| IBIS file usssdx1xxax.ibs created by s2ibis3 verion 1.1
| North Carolina State University, ERL, 2006
| This Model is valid for High-Rel grade Temperature Range -55C<=Tc<=125C
| Valid for DDR-333/400 operation
| Part Number   VDD/VDDQ   Package   Architecture
| SCB25D1G800AF   2.5 +0.2/-0.2  60-Ball FBGA   128Meg x 8
| SCB25D512800AF   2.5 +0.2/-0.2  60-Ball FBGA   64Meg x 8
| SCB25D1G160AF   2.5 +0.2/-0.2  60-Ball FBGA   64Meg x 16
| SCB25D1G160AE   2.5 +0.2/-0.2  66-Pin  Tsop   64Meg x 16
| SCB25D1G800AE   2.5 +0.2/-0.2  66-Pin  Tsop   128Meg x 8
| SCB25D512800AE   2.5 +0.2/-0.2  66-Pin  Tsop   64Meg x 8
| SCB25D512160AF   2.5 +0.2/-0.2  60-Ball FBGA   32Meg x 16
| SCB25D512160AE   2.5 +0.2/-0.2  66-Pin  Tsop   32Meg x 16
[IBIS Ver]   3.2
[File name]  usssdx1xxax.ibs
[File Rev]   1.2
[Date]   2016-10-27
[Source]   Simulation of a silicon level SPICE model
[Notes]   IBIS Characteristics for I/O Buffer
   IBIS Model Revision History:
Rev 1.1: 2015-10-27
   - IBIS model file initial creation
Rev 1.2: 2016-10-27
   - Updata company and other informations
   - Put components with different package into one IBIS model
[disclaimer] The IBIS models are for modeling purpose only and are
   subject to change without any notice. UniIC is not
   responsible for any problems the models may cause.
[Copyright]  Copyright 2009 UniIC Semiconductors Corp. All rights reserved
|   Component SCB25D1G800AF
[Component]   SCB25D1G800AF
[Manufacturer]  UniIC Semiconductors Corp.
| All balls excluding NC, POWER and GND (R[Ohm], L[H], C[F])
[Package]   |60-Ball FBGA
|Variable   typ   min   max
R_pkg   347m   219m   797m
L_pkg   1.51n   0.84n   3.21n
C_pkg   1.16p   0.74p   1.68p
[Pin]   signal_name model_name   R_pin   L_pin   C_pin
A1   VSSQ   GND
A2   DQ7   DQ   678m   2.88n   1.52p
A3   VSS   GND
A7   VDD   POWER
A8   DQ0   DQ   439m   1.68n   1.31p
A9   VDDQ   POWER
B2   VDDQ   POWER
B3   DQ6   DQ   797m   3.21n   1.68p
B7   DQ1   DQ   325m   1.24n   1.16p
B8   VSSQ   GND
C2   VSSQ   GND
C3   DQ5   DQ   476m   2.21n   1.25p
C7   DQ2   DQ   271m   0.99n   1.08p
C8   VDDQ   POWER
D2   VDDQ   POWER
D3   DQ4   DQ   395m   1.80n   1.16p
D7   DQ3   DQ   234m   0.84n   1.04p
D8   VSSQ   GND
E2   VSSQ   GND
E3   DQS   DQ   350m   1.48n   1.11p
E8   VDDQ   POWER
F1   VREF   POWER
F2   VSS   GND
F3   DM   DATA_RCV   299m   1.32n   1.04p
F8   VDD   POWER
F9   A5   CLKCA_RCV   314m   1.43n   1.13p
G2   CK   CLKCA_RCV   248m   1.16n   1.19p
G3   CK#   CLKCA_RCV   341m   1.59n   1.06p
G7   WE#   CLKCA_RCV   232m   1.10n   1.00p
G8   CAS#   CLKCA_RCV   340m   1.50n   1.18p
H2   A4   CLKCA_RCV   463m   1.90n   1.31p
H3   CKE   CLKCA_RCV   221m   1.03n   1.02p
H7   RAS#   CLKCA_RCV   219m   1.03n   1.01p
H8   CS#   CLKCA_RCV   318m   1.45n   1.14p
J2   A3   CLKCA_RCV   396m   1.83n   1.22p
J3   A13   CLKCA_RCV   438m   1.98n   1.29p
J7   BA1   CLKCA_RCV   242m   1.05n   1.06p
J8   BA0   CLKCA_RCV   357m   1.54n   1.21p
K2   A12   CLKCA_RCV   326m   1.52n   1.16p
K3   A11   CLKCA_RCV   340m   1.43n   1.18p
K7   A0   CLKCA_RCV   228m   1.03n   1.00p
K8   A2   CLKCA_RCV   264m   1.22n   1.08p
L2   A10   CLKCA_RCV   316m   1.49n   1.13p
L3   A9   CLKCA_RCV   236m   1.06n   1.02p
L7   A6   CLKCA_RCV   394m   1.66n   1.24p
L8   A1   CLKCA_RCV   344m   1.44n   1.19p
M2   A8   CLKCA_RCV   360m   1.57n   1.18p
M3   VSS   GND
M7   VDD   POWER
M8   A7   CLKCA_RCV   251m   1.04n   1.07p
|*****************************  Diff Pin  *************************************
[Diff Pin]  inv_pin  vdiff   tdelay_typ  tdelay_min  tdelay_max
G2   G3   0.62V   NA   NA   NA
|   Component SCB25D512800AF
[Component]   SCB25D512800AF
[Manufacturer]  UniIC Semiconductors Corp.
| All balls excluding NC, POWER and GND (R[Ohm], L[H], C[F])
[Package]   |60-Ball FBGA
|Variable   typ   min   max
R_pkg   347m   219m   797m
L_pkg   1.51n   0.84n   3.21n
C_pkg   1.16p   0.74p   1.68p
[Pin]   signal_name model_name   R_pin   L_pin   C_pin
A1   VSSQ   GND
A2   DQ7   DQ   678m   2.88n   1.52p
A3   VSS   GND
A7   VDD   POWER
A8   DQ0   DQ   439m   1.68n   1.31p
A9   VDDQ   POWER
B2   VDDQ   POWER
B3   DQ6   DQ   797m   3.21n   1.68p
B7   DQ1   DQ   325m   1.24n   1.16p
B8   VSSQ   GND
C2   VSSQ   GND
C3   DQ5   DQ   476m   2.21n   1.25p
C7   DQ2   DQ   271m   0.99n   1.08p
C8   VDDQ   POWER
D2   VDDQ   POWER
D3   DQ4   DQ   395m   1.80n   1.16p
D7   DQ3   DQ   234m   0.84n   1.04p
D8   VSSQ   GND
E2   VSSQ   GND
E3   DQS   DQ   350m   1.48n   1.11p
E8   VDDQ   POWER
F1   VREF   POWER
F2   VSS   GND
F3   DM   DATA_RCV   299m   1.32n   1.04p
F8   VDD   POWER
F9   A5   CLKCA_RCV   314m   1.43n   1.13p
G2   CK   CLKCA_RCV   248m   1.16n   1.19p
G3   CK#   CLKCA_RCV   341m   1.59n   1.06p
G7   WE#   CLKCA_RCV   232m   1.10n   1.00p
G8   CAS#   CLKCA_RCV   340m   1.50n   1.18p
H2   A4   CLKCA_RCV   463m   1.90n   1.31p
H3   CKE   CLKCA_RCV   221m   1.03n   1.02p
H7   RAS#   CLKCA_RCV   219m   1.03n   1.01p
H8   CS#   CLKCA_RCV   318m   1.45n   1.14p
J2   A3   CLKCA_RCV   396m   1.83n   1.22p
J3   A13   CLKCA_RCV   438m   1.98n   1.29p
J7   BA1   CLKCA_RCV   242m   1.05n   1.06p
J8   BA0   CLKCA_RCV   357m   1.54n   1.21p
K2   A12   CLKCA_RCV   326m   1.52n   1.16p
K3   A11   CLKCA_RCV   340m   1.43n   1.18p
K7   A0   CLKCA_RCV   228m   1.03n   1.00p
K8   A2   CLKCA_RCV   264m   1.22n   1.08p
L2   A10   CLKCA_RCV   316m   1.49n   1.13p
L3   A9   CLKCA_RCV   236m   1.06n   1.02p
L7   A6   CLKCA_RCV   394m   1.66n   1.24p
L8   A1   CLKCA_RCV   344m   1.44n   1.19p
M2   A8   CLKCA_RCV   360m   1.57n   1.18p
M3   VSS   GND
M7   VDD   POWER
M8   A7   CLKCA_RCV   251m   1.04n   1.07p
|*****************************  Diff Pin  *************************************
[Diff Pin]  inv_pin  vdiff   tdelay_typ  tdelay_min  tdelay_max
G2   G3   0.62V   NA   NA   NA
|   Component SCB25D1G160AF
[Component]   SCB25D1G160AF
[Manufacturer]  UniIC Semiconductors Corp.
| All balls excluding NC, POWER and GND (R[Ohm], L[H], C[F])
[Package]   |60-Ball FBGA
|Variable   typ   min   max
R_pkg   379m   230m   629m
L_pkg   1.71n   1.1n   2.4n
C_pkg   0.37p   0.21p   0.61p
[Pin]   signal_name model_name   R_pin   L_pin   C_pin
A1   VSSQ   GND
A2   DQ15   DQ   429m   1.6n   0.44p
A3   VSS   GND
A7   VDD   POWER
A8   DQ0   DQ   462m   1.78n   0.48p
A9   VDDQ   POWER
B1   DQ14   DQ   525m   2.04n   0.54p
B2   VDDQ   POWER
B3   DQ13   DQ   330m   1.41n   0.33p
B7   DQ2   DQ   361m   1.63n   0.38p
B8   VSSQ   GND
B9   DQ1   DQ   584m   2.26n   0.59p
C1   DQ12   DQ   539m   2.07n   0.54p
C2   VSSQ   GND
C3   DQ11   DQ   389m   1.67n   0.39p
C7   DQ4   DQ   366m   1.49n   0.37p
C9   DQ3   DQ   550m   2.36n   0.53p
D1   DQ10   DQ   629m   2.4n   0.61p
D2   VDDQ   POWER
D3   DQ9   DQ   356m   1.63n   0.36p
D7   DQ6   DQ   318m   1.45n   0.33p
D8   VSSQ   GND
D9   DQ5   DQ   556m   2.09n   0.54p
E1   DQ8   DQ   539m   2.18n   0.52p
E2   VSSQ   GND
E3   UDQS   DQ   307m   1.41n   0.3p
E7   LDQS   DQ   305m   1.27n   0.31p
E8   VDDQ   POWER
E9   DQ7   DQ   493m   2.32n   0.48p
F1   VREF   POWER
F2   VSS   GND
F3   UDM   DATA_RCV   235m   1.12n   0.23p
F7   LDM   DATA_RCV   254m   1.1n   0.27p
F8   VDD   POWER
F9   A13   CLKCA_RCV   480m   2.12n   0.44p
G2   CK   CLKCA_RCV   364m   1.98n   0.35p
G3   CK#   CLKCA_RCV   359m   1.78n   0.35p
G7   WE#   CLKCA_RCV   240m   1.23n   0.21p
G8   CAS#   CLKCA_RCV   350m   1.87n   0.32p
H2   A12   CLKCA_RCV   344m   1.82n   0.33p
H3   CKE   CLKCA_RCV   230m   1.21n   0.24p
H7   RAS#   CLKCA_RCV   231m   1.22n   0.22p
H8   CS#   CLKCA_RCV   341m   1.62n   0.31p
J2   A11   CLKCA_RCV   372m   1.72n   0.36p
J3   A9   CLKCA_RCV   257m   1.23n   0.26p
J7   BA1   CLKCA_RCV   269m   1.23n   0.28p
J8   BA0   CLKCA_RCV   421m   1.79n   0.42p
K2   A8   CLKCA_RCV   384m   1.95n   0.37p
K3   A7   CLKCA_RCV   274m   1.3n   0.28p
K7   A0   CLKCA_RCV   232m   1.19n   0.21p
K8   A10   CLKCA_RCV   342m   1.8n   0.31p
L2   A6   CLKCA_RCV   435m   1.95n   0.4p
L3   A5   CLKCA_RCV   317m   1.66n   0.3p
L7   A2   CLKCA_RCV   261m   1.39n   0.25p
L8   A1   CLKCA_RCV   362m   1.76n   0.33p
M2   A4   CLKCA_RCV   493m   2.13n   0.46p
M3   VSS   GND
M7   VDD   POWER
M8   A3   CLKCA_RCV   412m   2.26n   0.35p
|*****************************  Diff Pin  *************************************
[Diff Pin]  inv_pin  vdiff   tdelay_typ  tdelay_min  tdelay_max
G2   G3   0.62V   NA   NA   NA
|   Component SCB25D1G160AE
[Component]   SCB25D1G160AE
[Manufacturer]  UniIC Semiconductors Corp.
| All balls excluding NC, POWER and GND (R[Ohm], L[H], C[F])
[Package]   |66-pin TSOP
|Variable   typ   min   max
R_pkg   342m   278m   403m
L_pkg   5.44n   4.03n   7.63n
C_pkg   1.14p   0.53p   2.45p
[Pin]   signal_name model_name   R_pin   L_pin   C_pin
1   VDD   POWER
2   DQ0   DQ   380m   5.01nH   1.28pF
3   VDDQ   POWER
4   DQ1   DQ   380m   5.12nH   1.24pF
5   DQ2   DQ   380m   5.7nH   1.74pF
6   VSSQ   GND
7   DQ3   DQ   360m   5.23nH   1.11pF
8   DQ4   DQ   380m   4.84nH   1.7pF
9   VDDQ   POWER
10   DQ5   DQ   350m   4.5nH   0.9pF
11   DQ6   DQ   330m   4.96nH   1.8pF
12   VSSQ   GND
13   DQ7   DQ   290m   4.66nH   0.56pF
15   VDDQ   POWER
16   LDQS   DQ   350m   4.23nH   0.67pF
17   A13   CLKCA_RCV   290m   4.03nH   0.53pF
18   VDD   POWER
20   LDM   DATA_RCV   380m   5.18nH   0.71pF
21   WE#   CLKCA_RCV   300m   4.76nH   0.63pF
22   CAS#   CLKCA_RCV   290m   4.65nH   0.69pF
23   RAS#   CLKCA_RCV   300m   4.99nH   0.76pF
24   CS#   CLKCA_RCV   310m   5.19nH   0.75pF
26   BA0   CLKCA_RCV   320m   5.45nH   0.89pF
27   BA1   CLKCA_RCV   330m   5.63nH   1.09pF
28   A10   CLKCA_RCV   330m   5.95nH   1.17pF
29   A0   CLKCA_RCV   340m   6.1nH   1.22pF
30   A1   CLKCA_RCV   350m   6.02nH   1.23pF
31   A2   CLKCA_RCV   360m   6.19nH   1.26pF
32   A3   CLKCA_RCV   360m   5.85nH   1.27pF
33   VDD   POWER
34   VSS   GND
35   A4   CLKCA_RCV   360m   7.63nH   1.3pF
36   A5   CLKCA_RCV   370m   7.35nH   1.27pF
37   A6   CLKCA_RCV   350m   6.97nH   1.25pF
38   A7   CLKCA_RCV   340m   6.7nH   1.24pF
39   A8   CLKCA_RCV   340m   6.44nH   1.19pF
40   A9   CLKCA_RCV   360m   6.03nH   1.12pF
41   A11   CLKCA_RCV   350m   5.96nH   1.06pF
42   A12   CLKCA_RCV   330m   5.68nH   0.85pF
44   CKE   CLKCA_RCV   300m   5.12nH   0.7pF
45   CK   CLKCA_RCV   290m   4.88nH   0.7pF
46   CK#   CLKCA_RCV   280m   4.71nH   0.6pF
47   UDM   DATA_RCV   400m   5.11nH   1.09pF
48   VSS   GND
49   VREF   POWER
51   UDQS   DQ   310m   4.61nH   1.07pF
52   VSSQ   GND
54   DQ8   DQ   310m   4.37nH   0.57pF
55   VDDQ   POWER
56   DQ9   DQ   340m   4.65nH   1.99pF
57   DQ10   DQ   350m   4.85nH   0.9pF
58   VSSQ   GND
59   DQ11   DQ   400m   5.38nH   1.68pF
60   DQ12   DQ   350m   4.6nH   1.11pF
61   VDDQ   POWER
62   DQ13   DQ   380m   4.94nH   2.45pF
63   DQ14   DQ   360m   5.99nH   1.24pF
64   VSSQ   GND
65   DQ15   DQ   360m   7.02nH   1.96pF
66   VSS   GND
|*****************************  Diff Pin  *************************************
[Diff Pin]  inv_pin  vdiff   tdelay_typ  tdelay_min  tdelay_max
45   46   0.62V   NA   NA   NA
|   Component SCB25D1G800AE
[Component]   SCB25D1G800AE
[Manufacturer]  UniIC Semiconductors Corp.
| All balls excluding NC, POWER and GND (R[Ohm], L[H], C[F])
[Package]   |66-pin TSOP
|Variable   typ   min   max
R_pkg   340m   280m   400m
L_pkg   5.59n   4.03n   7.63n
C_pkg   1.20p   0.53p   2.45p
[Pin]   signal_name model_name   R_pin   L_pin   C_pin
1   VDD   POWER
2   DQ0   DQ   380m   5.01nH   1.28pF
3   VDDQ   POWER
5   DQ1   DQ   380m   5.7nH   1.74pF
6   VSSQ   GND
8   DQ2   DQ   380m   4.84nH   1.7pF
9   VDDQ   POWER
11   DQ3   DQ   330m   4.96nH   1.8pF
12   VSSQ   GND
15   VDDQ   POWER
17   A13   CLKCA_RCV   290m   4.03nH   0.53pF
18   VDD   POWER
21   WE#   CLKCA_RCV   300m   4.76nH   0.63pF
22   CAS#   CLKCA_RCV   290m   4.65nH   0.69pF
23   RAS#   CLKCA_RCV   300m   4.99nH   0.76pF
24   CS#   CLKCA_RCV   310m   5.19nH   0.75pF
26   BA0   CLKCA_RCV   320m   5.45nH   0.89pF
27   BA1   CLKCA_RCV   330m   5.63nH   1.09pF
28   A10   CLKCA_RCV   330m   5.95nH   1.17pF
29   A0   CLKCA_RCV   340m   6.1nH   1.22pF
30   A1   CLKCA_RCV   350m   6.02nH   1.23pF
31   A2   CLKCA_RCV   360m   6.19nH   1.26pF
32   A3   CLKCA_RCV   360m   5.85nH   1.27pF
33   VDD   POWER
34   VSS   GND
35   A4   CLKCA_RCV   360m   7.63nH   1.3pF
36   A5   CLKCA_RCV   370m   7.35nH   1.27pF
37   A6   CLKCA_RCV   350m   6.97nH   1.25pF
38   A7   CLKCA_RCV   340m   6.7nH   1.24pF
39   A8   CLKCA_RCV   340m   6.44nH   1.19pF
40   A9   CLKCA_RCV   360m   6.03nH   1.12pF
41   A11   CLKCA_RCV   350m   5.96nH   1.06pF
42   A12   CLKCA_RCV   330m   5.68nH   0.85pF
44   CKE   CLKCA_RCV   300m   5.12nH   0.7pF
45   CK   CLKCA_RCV   290m   4.88nH   0.7pF
46   CK#   CLKCA_RCV   280m   4.71nH   0.6pF
47   DM   DATA_RCV   400m   5.11nH   1.09pF
48   VSS   GND
49   VREF   POWER
51   DQS   DQ   310m   4.61nH   1.07pF
52   VSSQ   GND
55   VDDQ   POWER
56   DQ4   DQ   340m   4.65nH   1.99pF
58   VSSQ   GND
59   DQ5   DQ   400m   5.38nH   1.68pF
61   VDDQ   POWER
62   DQ6   DQ   380m   4.94nH   2.45pF
64   VSSQ   GND
65   DQ7   DQ   360m   7.02nH   1.96pF
66   VSS   GND
|*****************************  Diff Pin  *************************************
[Diff Pin]  inv_pin  vdiff   tdelay_typ  tdelay_min  tdelay_max
45   46   0.62V   NA   NA   NA
|   Component SCB25D512800AE
[Component]   SCB25D512800AE
[Manufacturer]  UniIC Semiconductors Corp.
| All balls excluding NC, POWER and GND (R[Ohm], L[H], C[F])
[Package]   |66-pin TSOP
|Variable   typ   min   max
R_pkg   340m   280m   400m
L_pkg   5.59n   4.03n   7.63n
C_pkg   1.20p   0.53p   2.45p
[Pin]   signal_name model_name   R_pin   L_pin   C_pin
1   VDD   POWER
2   DQ0   DQ   380m   5.01nH   1.28pF
3   VDDQ   POWER
5   DQ1   DQ   380m   5.7nH   1.74pF
6   VSSQ   GND
8   DQ2   DQ   380m   4.84nH   1.7pF
9   VDDQ   POWER
11   DQ3   DQ   330m   4.96nH   1.8pF
12   VSSQ   GND
15   VDDQ   POWER
17   A13   CLKCA_RCV   290m   4.03nH   0.53pF
18   VDD   POWER
21   WE#   CLKCA_RCV   300m   4.76nH   0.63pF
22   CAS#   CLKCA_RCV   290m   4.65nH   0.69pF
23   RAS#   CLKCA_RCV   300m   4.99nH   0.76pF
24   CS#   CLKCA_RCV   310m   5.19nH   0.75pF
26   BA0   CLKCA_RCV   320m   5.45nH   0.89pF
27   BA1   CLKCA_RCV   330m   5.63nH   1.09pF
28   A10   CLKCA_RCV   330m   5.95nH   1.17pF
29   A0   CLKCA_RCV   340m   6.1nH   1.22pF
30   A1   CLKCA_RCV   350m   6.02nH   1.23pF
31   A2   CLKCA_RCV   360m   6.19nH   1.26pF
32   A3   CLKCA_RCV   360m   5.85nH   1.27pF
33   VDD   POWER
34   VSS   GND
35   A4   CLKCA_RCV   360m   7.63nH   1.3pF
36   A5   CLKCA_RCV   370m   7.35nH   1.27pF
37   A6   CLKCA_RCV   350m   6.97nH   1.25pF
38   A7   CLKCA_RCV   340m   6.7nH   1.24pF
39   A8   CLKCA_RCV   340m   6.44nH   1.19pF
40   A9   CLKCA_RCV   360m   6.03nH   1.12pF
41   A11   CLKCA_RCV   350m   5.96nH   1.06pF
42   A12   CLKCA_RCV   330m   5.68nH   0.85pF
44   CKE   CLKCA_RCV   300m   5.12nH   0.7pF
45   CK   CLKCA_RCV   290m   4.88nH   0.7pF
46   CK#   CLKCA_RCV   280m   4.71nH   0.6pF
47   DM   DATA_RCV   400m   5.11nH   1.09pF
48   VSS   GND
49   VREF   POWER
51   DQS   DQ   310m   4.61nH   1.07pF
52   VSSQ   GND
55   VDDQ   POWER
56   DQ4   DQ   340m   4.65nH   1.99pF
58   VSSQ   GND
59   DQ5   DQ   400m   5.38nH   1.68pF
61   VDDQ   POWER
62   DQ6   DQ   380m   4.94nH   2.45pF
64   VSSQ   GND
65   DQ7   DQ   360m   7.02nH   1.96pF
66   VSS   GND
|*****************************  Diff Pin  *************************************
[Diff Pin]  inv_pin  vdiff   tdelay_typ  tdelay_min  tdelay_max
45   46   0.62V   NA   NA   NA
|   Component SCB25D512160AF
[Component]   SCB25D512160AF
[Manufacturer]  UniIC Semiconductors Corp.
| All balls excluding NC, POWER and GND (R[Ohm], L[H], C[F])
[Package]   |60-Ball FBGA
|Variable   typ   min   max
R_pkg   379m   230m   629m
L_pkg   1.71n   1.1n   2.4n
C_pkg   0.37p   0.21p   0.61p
[Pin]   signal_name model_name   R_pin   L_pin   C_pin
A1   VSSQ   GND
A2   DQ15   DQ   429m   1.6n   0.44p
A3   VSS   GND
A7   VDD   POWER
A8   DQ0   DQ   462m   1.78n   0.48p
A9   VDDQ   POWER
B1   DQ14   DQ   525m   2.04n   0.54p
B2   VDDQ   POWER
B3   DQ13   DQ   330m   1.41n   0.33p
B7   DQ2   DQ   361m   1.63n   0.38p
B8   VSSQ   GND
B9   DQ1   DQ   584m   2.26n   0.59p
C1   DQ12   DQ   539m   2.07n   0.54p
C2   VSSQ   GND
C3   DQ11   DQ   389m   1.67n   0.39p
C7   DQ4   DQ   366m   1.49n   0.37p
C9   DQ3   DQ   550m   2.36n   0.53p
D1   DQ10   DQ   629m   2.4n   0.61p
D2   VDDQ   POWER
D3   DQ9   DQ   356m   1.63n   0.36p
D7   DQ6   DQ   318m   1.45n   0.33p
D8   VSSQ   GND
D9   DQ5   DQ   556m   2.09n   0.54p
E1   DQ8   DQ   539m   2.18n   0.52p
E2   VSSQ   GND
E3   UDQS   DQ   307m   1.41n   0.3p
E7   LDQS   DQ   305m   1.27n   0.31p
E8   VDDQ   POWER
E9   DQ7   DQ   493m   2.32n   0.48p
F1   VREF   POWER
F2   VSS   GND
F3   UDM   DATA_RCV   235m   1.12n   0.23p
F7   LDM   DATA_RCV   254m   1.1n   0.27p
F8   VDD   POWER
G2   CK   CLKCA_RCV   364m   1.98n   0.35p
G3   CK#   CLKCA_RCV   359m   1.78n   0.35p
G7   WE#   CLKCA_RCV   240m   1.23n   0.21p
G8   CAS#   CLKCA_RCV   350m   1.87n   0.32p
H2   A12   CLKCA_RCV   344m   1.82n   0.33p
H3   CKE   CLKCA_RCV   230m   1.21n   0.24p
H7   RAS#   CLKCA_RCV   231m   1.22n   0.22p
H8   CS#   CLKCA_RCV   341m   1.62n   0.31p
J2   A11   CLKCA_RCV   372m   1.72n   0.36p
J3   A9   CLKCA_RCV   257m   1.23n   0.26p
J7   BA1   CLKCA_RCV   269m   1.23n   0.28p
J8   BA0   CLKCA_RCV   421m   1.79n   0.42p
K2   A8   CLKCA_RCV   384m   1.95n   0.37p
K3   A7   CLKCA_RCV   274m   1.3n   0.28p
K7   A0   CLKCA_RCV   232m   1.19n   0.21p
K8   A10   CLKCA_RCV   342m   1.8n   0.31p
L2   A6   CLKCA_RCV   435m   1.95n   0.4p
L3   A5   CLKCA_RCV   317m   1.66n   0.3p
L7   A2   CLKCA_RCV   261m   1.39n   0.25p
L8   A1   CLKCA_RCV   362m   1.76n   0.33p
M2   A4   CLKCA_RCV   493m   2.13n   0.46p
M3   VSS   GND
M7   VDD   POWER
M8   A3   CLKCA_RCV   412m   2.26n   0.35p
|*****************************  Diff Pin  *************************************
[Diff Pin]  inv_pin  vdiff   tdelay_typ  tdelay_min  tdelay_max
G2   G3   0.62V   NA   NA   NA
|   Component SCB25D512160AE
[Component]   SCB25D512160AE
[Manufacturer]  UniIC Semiconductors Corp.
| All balls excluding NC, POWER and GND (R[Ohm], L[H], C[F])
[Package]   |66-pin TSOP
|Variable   typ   min   max
R_pkg   379m   230m   629m
L_pkg   1.71n   1.1n   2.4n
C_pkg   0.37p   0.21p   0.61p
[Pin]   signal_name model_name   R_pin   L_pin   C_pin
1   VDD   POWER
2   DQ0   DQ   380m   5.01nH   1.28pF
3   VDDQ   POWER
4   DQ1   DQ   380m   5.12nH   1.24pF
5   DQ2   DQ   380m   5.7nH   1.74pF
6   VSSQ   GND
7   DQ3   DQ   360m   5.23nH   1.11pF
8   DQ4   DQ   380m   4.84nH   1.7pF
9   VDDQ   POWER
10   DQ5   DQ   350m   4.5nH   0.9pF
11   DQ6   DQ   330m   4.96nH   1.8pF
12   VSSQ   GND
13   DQ7   DQ   290m   4.66nH   0.56pF
15   VDDQ   POWER
16   LDQS   CLKCA_RCV   350m   4.23nH   0.67pF
18   VDD   POWER
20   LDM   DATA_RCV   380m   5.18nH   0.71pF
21   WE#   CLKCA_RCV   300m   4.76nH   0.63pF
22   CAS#   CLKCA_RCV   290m   4.65nH   0.69pF
23   RAS#   CLKCA_RCV   300m   4.99nH   0.76pF
24   CS#   CLKCA_RCV   310m   5.19nH   0.75pF
26   BA0   CLKCA_RCV   320m   5.45nH   0.89pF
27   BA1   CLKCA_RCV   330m   5.63nH   1.09pF
28   A10   CLKCA_RCV   330m   5.95nH   1.17pF
29   A0   CLKCA_RCV   340m   6.1nH   1.22pF
30   A1   CLKCA_RCV   350m   6.02nH   1.23pF
31   A2   CLKCA_RCV   360m   6.19nH   1.26pF
32   A3   CLKCA_RCV   360m   5.85nH   1.27pF
33   VDD   POWER
34   VSS   GND
35   A4   CLKCA_RCV   360m   7.63nH   1.3pF
36   A5   CLKCA_RCV   370m   7.35nH   1.27pF
37   A6   CLKCA_RCV   350m   6.97nH   1.25pF
38   A7   CLKCA_RCV   340m   6.7nH   1.24pF
39   A8   CLKCA_RCV   340m   6.44nH   1.19pF
40   A9   CLKCA_RCV   360m   6.03nH   1.12pF
41   A11   CLKCA_RCV   350m   5.96nH   1.06pF
42   A12   CLKCA_RCV   330m   5.68nH   0.85pF
44   CKE   CLKCA_RCV   300m   5.12nH   0.7pF
45   CK   CLKCA_RCV   290m   4.88nH   0.7pF
46   CKB   CLKCA_RCV   280m   4.71nH   0.6pF
47   UDM   DATA_RCV   400m   5.11nH   1.09pF
48   VSS   GND
49   VREF   POWER
51   UDQS   CLKCA_RCV   310m   4.61nH   1.07pF
52   VSSQ   GND
54   DQ8   DQ   310m   4.37nH   0.57pF
55   VDDQ   POWER
56   DQ9   DQ   340m   4.65nH   1.99pF
57   DQ10   DQ   350m   4.85nH   0.9pF
58   VSSQ   GND
59   DQ11   DQ   400m   5.38nH   1.68pF
60   DQ12   DQ   350m   4.6nH   1.11pF
61   VDDQ   POWER
62   DQ13   DQ   380m   4.94nH   2.45pF
63   DQ14   DQ   360m   5.99nH   1.24pF
64   VSSQ   GND
65   DQ15   DQ   360m   7.02nH   1.96pF
66   VSS   GND
|*****************************  Diff Pin  *************************************
[Diff Pin]  inv_pin  vdiff   tdelay_typ  tdelay_min  tdelay_max
45   46   0.62V   NA   NA   NA
|*****************************  Model Selector ********************************
[Model Selector]   DQ
DATA_FULL   Full-Strength Output Driver
DATA_HALF   Weak Strength Output Driver
DATA_RCV   Data/Data Strobe/Data Mask Receiver
| Models and submodels in the file (4): DATA_FULL (I/O), DATA_HALF (I/O), DATA_RCV (Input), CLKCA_RCV (Input)
